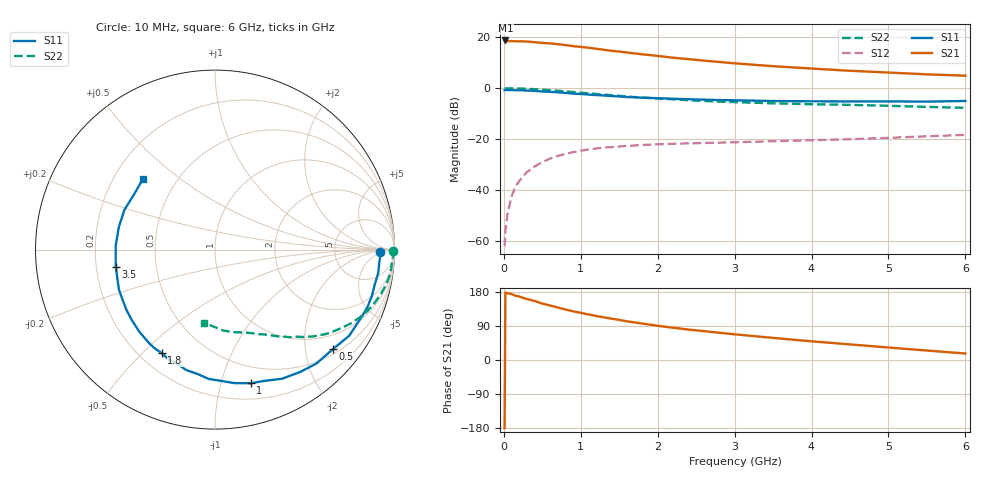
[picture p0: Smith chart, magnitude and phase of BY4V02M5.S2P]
! SIEMENS Small Signal Semiconductors
! BFY420
! Si NPN RF SIEGET Grounded Emitter Transistor in MICRO-X
! VCE = 4 V  IC = 2.5 mA
! Common Emitter S-Parameters:  October  1996
# GHz  S  MA  R  50
!  f  S11  S21  S12  S22
! GHz  MAG  ANG  MAG  ANG  MAG  ANG  MAG  ANG
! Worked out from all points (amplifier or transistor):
!   36 points, 10 MHz to 6 GHz, reference 50 ohm
!   highest |S21| = 18.7 dB at 20 MHz (marker M1)
!   |S21| within 3 dB of that: start of sweep to 1.139 GHz
!   unconditionally stable (mu >= 1): 3.811 GHz to end of sweep
!   at 250 MHz: K = 0.09, MSG = 26.4 dB, |S12| = -34.5 dB
!   at 1.4 GHz: K = 0.34, MSG = 18.9 dB, |S12| = -23.1 dB
!   at 6 GHz: K = 1.20, MAG = 8.9 dB, |S12| = -18.3 dB
!   S11 on the Smith chart (normalised r, x): 10 MHz: 23, -4; 500 MHz: 0.61, -2.61; 1 GHz: 0.34, -1.25; 1.8 GHz: 0.29, -0.57; 3.5 GHz: 0.28, -0.08; 6 GHz: 0.32, +0.37
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0.01  0.9172 -0.8  8.578 -179.8  0.0008 51.5  0.994 -0.4
0.02  0.9226 -2.1  8.632 178.1  0.0016 69.0  0.9869 -0.8
0.05  0.9185 -4.1  8.375 176.1  0.0036 86.6  0.9934 -1.9
0.1  0.9186 -8.3  8.374 173.9  0.0075 82.4  0.9883 -3.9
0.15  0.9111 -12.4  8.326 169.7  0.0117 78.6  0.9876 -5.9
0.2  0.9114 -16.5  8.297 167.5  0.0151 78.6  0.9846 -7.7
0.3  0.8987 -24.7  8.211 160.9  0.0226 75.3  0.973 -11.5
0.4  0.8883 -32.7  7.99 155.7  0.0292 70.8  0.9561 -15.2
0.5  0.8597 -40.2  7.724 148.9  0.0355 66.8  0.9367 -18.6
0.7  0.8302 -55.3  7.317 138.6  0.0469 59.8  0.8908 -25.1
0.8  0.8107 -62.6  7.008 133.3  0.0516 55.7  0.8655 -28.1
1  0.7706 -75.0  6.436 124.4  0.0594 50.2  0.8169 -33.0
1.1  0.752 -81.7  6.222 120.2  0.063 47.6  0.7944 -35.5
1.4  0.7 -97.9  5.408 109.0  0.0699 40.9  0.7301 -41.5
1.6  0.6705 -108.4  5.002 102.1  0.0741 37.4  0.6888 -45.0
1.8  0.6493 -117.2  4.613 96.1  0.0768 34.5  0.6567 -47.8
2.2  0.6218 -132.8  3.963 85.2  0.0813 30.1  0.6052 -53.3
2.8  0.5854 -151.9  3.274 71.9  0.0858 26.1  0.5452 -60.0
3.5  0.5611 -170.3  2.702 58.3  0.0912 24.0  0.5052 -66.9
4.5  0.5505 166.9  2.196 41.2  0.1002 22.4  0.4711 -77.6
5.5  0.546 145.5  1.869 25.0  0.1141 21.0  0.4299 -90.8
6  0.5616 135.9  1.758 17.1  0.1218 19.7  0.4127 -98.5
